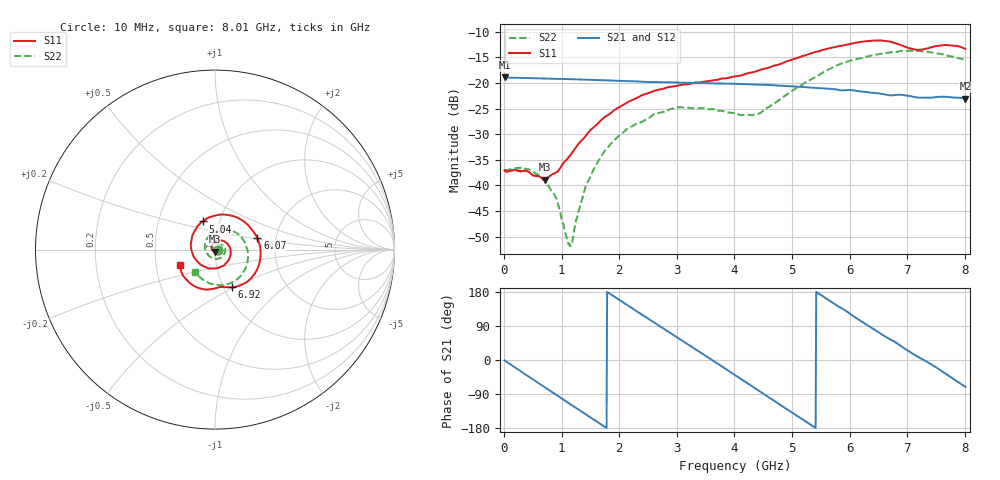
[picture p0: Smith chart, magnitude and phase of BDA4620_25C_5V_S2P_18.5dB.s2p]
!Agilent Technologies,E5071B,MY42404982,A.09.10
!Date: Wed May 06 09:02:14 2026
!Data & Calibration Information:
!Freq	S11:SOLT2(ON)	S21:SOLT2(ON)	S12:SOLT2(ON)	S22:SOLT2(ON)
# Hz S RI R 50
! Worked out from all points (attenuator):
!   801 points, 10 MHz to 8.01 GHz, reference 50 ohm
!   highest |S21| = -18.91 dB at 10 MHz (marker M1); lowest = -23.1 dB at 8.01 GHz (marker M2)
!   lowest |S11| = -38.9 dB at 710 MHz (marker M3), VSWR 1.02, Z = 49.7 - j1.09 ohm
!   |S11| at or under -10 dB: start of sweep to end of sweep
!   |S22| runs from -51.9 to -13.7 dB; largest |S21 - S12| = 0.00051
!   S11 on the Smith chart (normalised r, x): 10 MHz: 1.03, -0.00; 5.04 GHz: 0.83, +0.27; 6.07 GHz: 1.60, +0.22; 6.92 GHz: 1.10, -0.49; 8.01 GHz: 0.66, -0.12
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1e7  0.014 -0.000918  0.1133 -0.0024  0.1134 -0.00242  0.014 -0.000499
4.4e8  0.00818 -0.0106  0.0789 -0.0788  0.079 -0.079  0.0132 -0.00534
7.1e8  -0.00274 -0.011  0.0337 -0.1053  0.0337 -0.1055  0.00813 -0.00741
9e8  -0.0112 -0.00728  -0.00268 -0.1098  -0.00273 -0.11  0.00328 -0.00687
1.14e9  -0.0186 0.00514  -0.0468 -0.0983  -0.047 -0.0984  -0.00221 -0.00151
1.19e9  -0.0193 0.00869  -0.0552 -0.0936  -0.0553 -0.0937  -0.0029 0.000174
1.35e9  -0.0192 0.0198  -0.0783 -0.0743  -0.0785 -0.0744  -0.00456 0.00548
1.58e9  -0.0111 0.0361  -0.1001 -0.0375  -0.1002 -0.0376  -0.00373 0.0147
1.86e9  0.0107 0.05  -0.1049 0.0134  -0.1049 0.0134  0.00402 0.0253
2.16e9  0.0424 0.0499  -0.0832 0.063  -0.0832 0.0631  0.0189 0.0308
2.68e9  0.0857 0.00309  -0.00325 0.1018  -0.00318 0.1019  0.0469 0.0191
3.07e9  0.0777 -0.0559  0.0603 0.081  0.0605 0.081  0.0574 -0.00859
4.01e9  -0.0809 -0.0825  0.0751 -0.0627  0.0752 -0.0629  -0.0135 -0.0486
4.42e9  -0.1325 0.00197  0.0157 -0.0948  0.0156 -0.0949  -0.0486 -0.0124
5.04e9  -0.0685 0.1571  -0.0734 -0.0561  -0.0736 -0.0561  -0.0283 0.0816
5.35e9  0.0249 0.1947  -0.0891 -0.0102  -0.0893 -0.0103  0.0241 0.1068
6.07e9  0.2359 0.0644  -0.0362 0.0763  -0.0362 0.0764  0.1615 0.0479
6.38e9  0.2498 -0.0646  0.00702 0.08  0.00703 0.08  0.1838 -0.0214
6.68e9  0.1815 -0.1775  0.0418 0.0633  0.0419 0.0634  0.1728 -0.0953
6.92e9  0.0957 -0.21  0.0635 0.0424  0.0636 0.0425  0.1416 -0.1488
7.57e9  -0.0796 -0.2172  0.0656 -0.0327  0.0659 -0.0326  -0.021 -0.1909
8.01e9  -0.1956 -0.088  0.0229 -0.0663  0.0231 -0.0666  -0.1091 -0.1262
